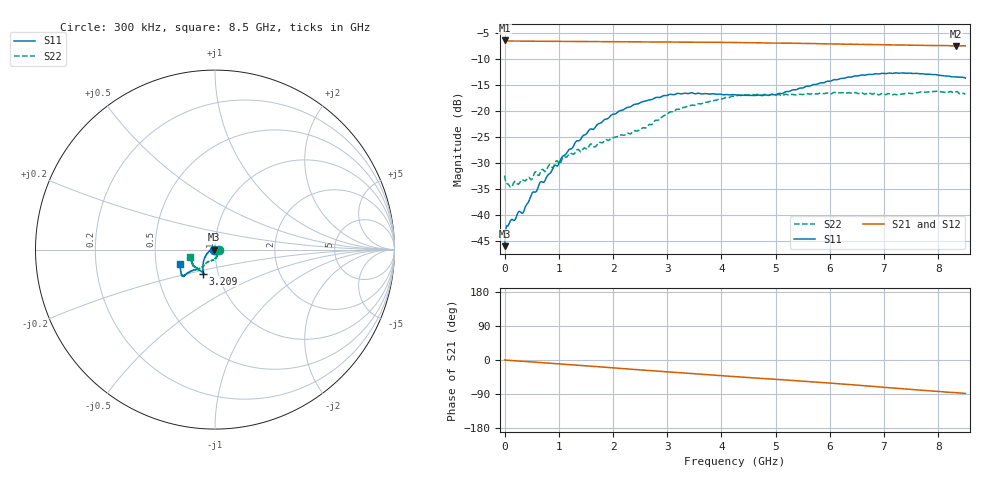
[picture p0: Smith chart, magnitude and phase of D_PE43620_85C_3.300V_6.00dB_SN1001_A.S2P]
! device id: pe43620
! dir: c:\dsa\pe43620\data\pe43620\085c\3p300v\06p00db
! Serial: 1001
! Insertion: A
! Temp: 85C
! VDD: 3.300V
! Attenuation Step: 6.00dB
! IDD: 9.746512e-03mA
! FILE NAME
! DATE 10-22-2008 15:09:15
! CORRECTED  DATA
#  Hz  S  RI  R  50.00
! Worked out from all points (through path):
!   401 points, 300 kHz to 8.5 GHz, reference 50 ohm
!   highest |S21| = -6.35 dB at 300 kHz (marker M1); lowest = -7.4 dB at 8.33 GHz (marker M2)
!   group delay of S21, straight-line fit = 28.6 ps
!   lowest |S11| = -45.9 dB at 300 kHz (marker M3), VSWR 1.01, Z = 49.5 - j0.0275 ohm
!   |S11| at or under -10 dB: start of sweep to end of sweep
!   |S22| runs from -34.6 to -16.1 dB; largest |S21 - S12| = 0.0023
!   S11 on the Smith chart (normalised r, x): 300 kHz: 0.99, -0.00; 3.209 GHz: 0.85, -0.23; 8.5 GHz: 0.67, -0.11
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300000  -0.00504 -0.000278  0.4812 -0.000886  0.4801 -0.000693  0.0241 -0.000694
6.404775e7  -0.00789 -0.000578  0.4754 -0.00644  0.4756 -0.00647  0.0197 -0.00306
8.5297e7  -0.00839 -0.000322  0.475 -0.00844  0.4748 -0.00827  0.0191 -0.00329
2.55291e8  -0.0108 0.000782  0.4741 -0.0219  0.4742 -0.022  0.0184 -0.00756
3.40288e8  -0.0106 0.000549  0.4736 -0.0287  0.4737 -0.029  0.0192 -0.0104
5.10282e8  -0.0165 0.00065  0.4717 -0.0428  0.4721 -0.043  0.0166 -0.0149
6.590268e8  -0.0209 -0.00165  0.4699 -0.0552  0.4702 -0.055  0.0167 -0.0197
7.440238e8  -0.0214 -0.00245  0.469 -0.062  0.4693 -0.0622  0.0156 -0.0212
1.190258e9  -0.0391 -0.018  0.461 -0.099  0.4614 -0.0993  0.0121 -0.037
1.424e9  -0.0486 -0.0281  0.4559 -0.1188  0.456 -0.119  0.00811 -0.0406
1.572745e9  -0.054 -0.0403  0.4519 -0.1311  0.4524 -0.131  0.0048 -0.0475
1.99773e9  -0.064 -0.0686  0.4383 -0.1657  0.4394 -0.1654  -0.00394 -0.0559
2.465213e9  -0.0671 -0.0974  0.4214 -0.2028  0.4214 -0.203  -0.022 -0.0616
2.8477e9  -0.0654 -0.1193  0.4052 -0.2306  0.4055 -0.2303  -0.0438 -0.0707
3.208937e9  -0.0654 -0.1337  0.3882 -0.2551  0.388 -0.2568  -0.0573 -0.0875
4.25015e9  -0.0727 -0.1245  0.3311 -0.3185  0.331 -0.3188  -0.0885 -0.1088
4.993874e9  -0.0952 -0.1084  0.2868 -0.3518  0.2854 -0.3526  -0.0964 -0.1046
5.67385e9  -0.1336 -0.1198  0.2402 -0.3789  0.2405 -0.3795  -0.113 -0.0956
6.460072e9  -0.1671 -0.142  0.1803 -0.4033  0.1814 -0.4037  -0.1262 -0.0844
7.09755e9  -0.1806 -0.1487  0.1269 -0.4183  0.1262 -0.4182  -0.1313 -0.0675
8.330006e9  -0.1941 -0.091  0.0273 -0.4255  0.0266 -0.4261  -0.1473 -0.0465
8.5e9  -0.1925 -0.0809  0.0144 -0.4269  0.0139 -0.4275  -0.1406 -0.0409
